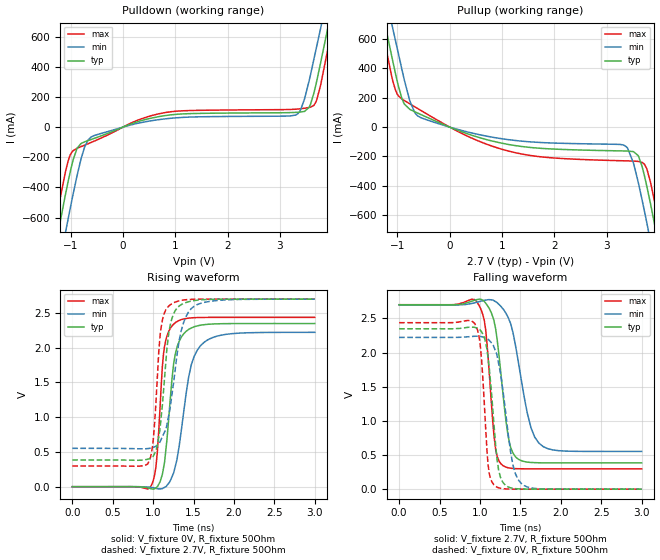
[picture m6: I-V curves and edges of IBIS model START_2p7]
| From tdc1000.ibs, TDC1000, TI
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|   Model
[Model]   START_2p7
Model_type   Output
Polarity   Non-Inverting
Vmeas = 1.35
Vref = 0
Cref = 1pF
Rref = 100000
|   typ   min   max
C_comp   3.839pF   2.875pF   5.918pF
[Voltage Range]   2.7   2.699   2.701
[Temperature Range]   27   125   -40
[Pullup Reference]   2.7   2.699   2.701
[Pulldown Reference]   0   0   0
[Power Clamp Reference]   2.7   2.699   2.701
[GND Clamp Reference]   0   0   0
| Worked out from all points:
|   slope of the pulldown table from 0 to 0.405 V, typ, clamps not added: 8.44 ohm
|   slope of the pullup table from 0 to 0.405 V, typ, clamps not added: 7.6 ohm
|   falling waveform, V_fixture 2.7V, R_fixture 50Ohm: 20-80 % time 133ps typ, 201ps min, 94.2ps max; typ from 2.7 V to 0.385 V
|   rising waveform, V_fixture 0V, R_fixture 50Ohm: 20-80 % time 118ps typ, 176ps min, 81.6ps max; typ from 0 V to 2.35 V
|   rising waveform, V_fixture 2.7V, R_fixture 50Ohm: 20-80 % time 111ps typ, 168ps min, 81.5ps max; typ from 0.385 V to 2.7 V
|   falling waveform, V_fixture 0V, R_fixture 50Ohm: 20-80 % time 104ps typ, 153ps min, 76.1ps max; typ from 2.35 V to 0 V
[Pulldown]
|   Voltage   I(typ)   I(min)   I(max)
-2.7V     -3.424A    -3.626A    -3.297A
-1.372V   -943.8mA   -1.199A    -780.5mA
-1.291V   -792.9mA   -1.051A    -630mA
-1.088V   -429.1mA   -681.8mA   -281.5mA
-877.5mV  -141.1mA   -323.1mA   -140.4mA
-731.7mV  -97.36mA   -131.4mA   -119.5mA
-610.2mV  -82.25mA   -66.2mA    -101.9mA
823.5mV   77.34mA    55.54mA    97.48mA
3.302V    97.88mA    80.1mA     119.1mA
3.561V    131.6mA    308.4mA    130.4mA
3.78V     426.2mA    655mA      277.4mA
5.4V      3.155A     3.26A      3.092A
[Pullup]
|   Voltage   I(typ)   I(min)   I(max)
-2.7V     3.166A     3.267A     3.108A
-1.104V   473.5mA    694.9mA    335.5mA
-885.6mV  169.2mA    346.3mA    185.1mA
-618.3mV  96.35mA    77.82mA    127.6mA
1.139V    -119.1mA   -86.07mA   -164.5mA
3.326V    -162.2mA   -122.6mA   -229.3mA
3.61V     -199.3mA   -385.7mA   -234mA
3.772V    -410.2mA   -659.7mA   -288.9mA
3.837V    -519.7mA   -775.6mA   -373.7mA
4.007V    -826.4mA   -1.086A    -664.8mA
4.104V    -1.008A    -1.263A    -844.5mA
5.4V      -3.426A    -3.631A    -3.299A
[Ramp]
R_load = 50
|   typ   min   max
dV/dt_r   1.40917/1.17645e-10   1.33312/1.76306e-10   1.46252/8.15883e-11
dV/dt_f   1.3892/1.32544e-10   1.28812/2.01432e-10   1.44203/9.41743e-11
[Falling Waveform]
V_fixture = 2.7V
V_fixture_min = 2.699V
V_fixture_max = 2.701V
R_fixture = 50Ohm
C_fixture = 0F
|   Time   V(typ)   V(min)   V(max)
0s        2.7V       2.699V     2.701V
968.3ps   2.778V     2.739V     2.731V
1.07ns    2.723V     2.768V     2.338V
1.171ns   2.478V     2.761V     809.8mV
1.283ns   1.414V     2.642V     345.9mV
1.349ns   771.6mV    2.515V     312.8mV
1.409ns   525.2mV    2.288V     303.3mV
1.585ns   397.1mV    1.117V     297.9mV
1.728ns   386.6mV    674.6mV    297.7mV
3ns       384.7mV    552.1mV    297.6mV
[Rising Waveform]
V_fixture = 0V
V_fixture_min = 0V
V_fixture_max = 0V
R_fixture = 50Ohm
C_fixture = 0F
|   Time   V(typ)   V(min)   V(max)
0s        -7.713uV   35.12uV    191.3pV
968.3ps   -27.8mV    -9.514mV   -691.9uV
1.034ns   -18.72mV   -23.51mV   276.9mV
1.115ns   177.3mV    -26.29mV   1.73V
1.172ns   691.6mV    19.32mV    2.172V
1.232ns   1.534V     138.7mV    2.311V
1.283ns   1.948V     332.8mV    2.368V
1.473ns   2.285V     1.756V     2.43V
1.631ns   2.332V     2.078V     2.437V
3ns       2.349V     2.222V     2.438V
[Rising Waveform]
V_fixture = 2.7V
V_fixture_min = 2.699V
V_fixture_max = 2.701V
R_fixture = 50Ohm
C_fixture = 0F
|   Time   V(typ)   V(min)   V(max)
0s        384.7mV    552.1mV    297.6mV
934.7ps   396.1mV    549.2mV    326.8mV
1ns       436.8mV    563.9mV    653.1mV
1.06ns    635.1mV    601.6mV    1.734V
1.114ns   1.168V     718.4mV    2.394V
1.171ns   1.993V     895.3mV    2.571V
1.213ns   2.333V     1.159V     2.62V
1.349ns   2.621V     2.251V     2.682V
1.507ns   2.679V     2.597V     2.698V
3ns       2.7V       2.699V     2.701V
[Falling Waveform]
|Gnd
V_fixture = 0V
V_fixture_min = 0V
V_fixture_max = 0V
R_fixture = 50Ohm
C_fixture = 0F
|   Time   V(typ)   V(min)   V(max)
0s        2.349V     2.222V     2.438V
934.7ps   2.369V     2.239V     2.427V
1.007ns   2.322V     2.236V     2.064V
1.087ns   2.05V      2.203V     567mV
1.129ns   1.597V     2.16V      162.2mV
1.194ns   644.9mV    2.018V     41mV
1.275ns   116.4mV    1.518V     8.783mV
1.407ns   12.63mV    358.2mV    813.7uV
1.507ns   2.939mV    87.11mV    133.9uV
3ns       10.61uV    35.25uV    -3.877nV
